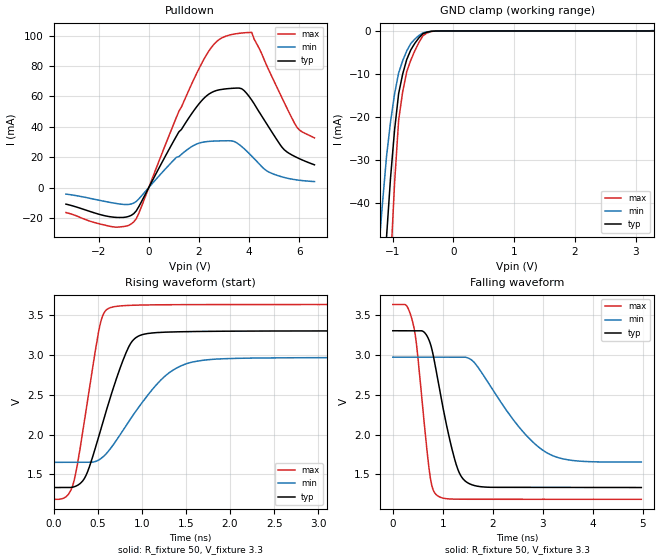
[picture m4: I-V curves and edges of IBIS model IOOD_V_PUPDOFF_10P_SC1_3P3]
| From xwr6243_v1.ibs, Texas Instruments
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|   Model Cell IOOD_V_PUPDOFF_10P_SC1_3P3
|IOOD_V_PUPDOFF_10P_SC1_3P3
[Model]   IOOD_V_PUPDOFF_10P_SC1_3P3
Model_type   I/O_open_drain
Polarity   Non-Inverting
Enable   Active-Low
Vinl =  0.8V
Vinh =  2V
Cref =  15pF
Rref =  100.0000M
Vref =  0V
Vmeas =  1.65
|   typ   min   max
C_comp   2.059994p   1.912853p   2.135747p
[Model Spec]
Vinl   0.8V   0.8V   0.8V
Vinh   2V   2V   2V
[Temperature Range]   25   125   -40
[Voltage Range]   3.3   2.97   3.63
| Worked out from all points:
|   slope of the pulldown table from 0 to 0.495 V, typ, clamps not added: 31.8 ohm
|   GND clamp passes 1 mA (typ) near -0.53 V on its own axis
|   rising waveform, R_fixture 50, V_fixture 3.3: 20-80 % time 334ps typ, 531ps min, 209ps max; typ from 1.34 V to 3.3 V
|   falling waveform, R_fixture 50, V_fixture 3.3: 20-80 % time 385ps typ, 931ps min, 234ps max; typ from 3.3 V to 1.34 V
| Where Nom  PVT is Nominal Process, 3.3V, 25C
|   Fast PVT is Strong Process,  3.63V, -40C
|   Slow PVT is Weak Process,   2.97V, 125C
[Pulldown]
|   voltage   I(typ)   I(min)   I(max)
-3.3V     -10.93mA   -4.311mA   -16.48mA
-1.4V     -19.53mA   -10.23mA   -25.96mA
-600mV    -17.23mA   -10.26mA   -22.66mA
1.1V      33.82mA    19.89mA    46.25mA
2V        55.14mA    29.24mA    78.29mA
2.6V      63.35mA    30.61mA    94.45mA
3.2V      65.21mA    30.81mA    100.4mA
3.7V      65.09mA    27.02mA    101.8mA
4.1V      57.63mA    20.71mA    102.2mA
5.3V      26.68mA    7.058mA    59.31mA
5.9V      19.77mA    5.007mA    39.76mA
6.6V      14.97mA    3.923mA    32.7mA
[GND_clamp]
|   voltage   I(typ)   I(min)   I(max)
-3.3V     -787.2mA   -607.8mA   -1.235A
-1.233V   -85.66mA   -52.14mA   -138.8mA
-1.167V   -66.47mA   -40.37mA   -107.7mA
-1.1V     -48.25mA   -29.37mA   -77.98mA
-1.033V   -34.27mA   -21.19mA   -54.56mA
-966.7mV  -23.06mA   -14.66mA   -35.51mA
-900mV    -14.61mA   -9.789mA   -20.83mA
-833.3mV  -10.05mA   -6.934mA   -14.15mA
-700mV    -4.416mA   -2.931mA   -6.811mA
-500mV    -621.6uA   -443.4uA   -1.094mA
-300mV    -17.13uA   -24.29uA   -23.57uA
3.3V      4.589uA    110.6uA    5.608uA
[Ramp]
| variable   typ   min   max
dV/dt_f  1.1805738/0.3856329n 0.79476876/0.93922811n  1.4675033/0.23410022n
dV/dt_r  1.1742366/0.46733719n 0.80289248/1.0812442n  1.4769635/0.2448637n
R_load = 50
[Rising Waveform]
R_fixture = 50
V_fixture = 3.3
V_fixture_min = 2.97
V_fixture_max = 3.63
|   time   V(typ)   V(min)   V(max)
0s        1.337V     1.652V     1.189V
223.4ps   1.343V     1.652V     1.383V
365.8ps   1.483V     1.652V     2.284V
518.8ps   2.001V     1.685V     3.334V
629.3ps   2.414V     1.802V     3.584V
806.8ps   2.985V     2.086V     3.616V
923.7ps   3.206V     2.279V     3.621V
1.266ns   3.283V     2.734V     3.627V
1.558ns   3.291V     2.904V     3.628V
4.974ns   3.3V       2.967V     3.63V
[Falling Waveform]
R_fixture = 50
V_fixture = 3.3
V_fixture_min = 2.97
V_fixture_max = 3.63
|   time   V(typ)   V(min)   V(max)
0s        3.3V       2.969V     3.629V
269.7ps   3.3V       2.969V     3.617V
405.9ps   3.3V       2.969V     3.388V
482.3ps   3.3V       2.969V     3.083V
737.7ps   3.161V     2.969V     1.513V
888ps     2.729V     2.969V     1.236V
1.25ns    1.664V     2.969V     1.19V
1.51ns    1.391V     2.958V     1.189V
3.071ns   1.337V     1.776V     1.188V
4.974ns   1.336V     1.656V     1.188V
